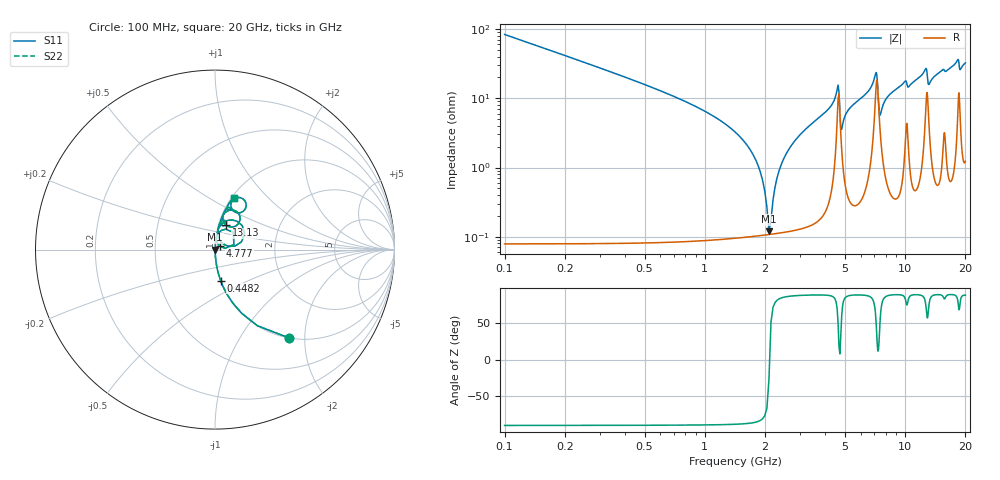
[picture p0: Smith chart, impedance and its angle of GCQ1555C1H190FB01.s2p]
!Murata Part Number: GCQ1555C1H190FB01
!These Parameters are Measured in Series Mode Connection
!Data Generated on Mar 13, 2026
!  o--ll--o
!Port1  Port2
!  o------o
!Operation Temp=25[degC], DC Bias Voltage=0[V]
!Freq. Start=100[MHz] Stop=20[GHz] 401[Steps]
# Hz S RI R 50
!Freq.(Hz) S11(Real) S11(Imag) S21(Real) S21(Imag) S12(Real) S12(Imag) S22(Real) S22(Imag)
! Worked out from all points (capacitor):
!   401 points, 100 MHz to 20 GHz, reference 50 ohm
!   read as one part in series: C = 19 pF near 199.5 MHz
!   lowest |Z| = 120 mohm at 2.09 GHz (marker M1)
!   series resonance near 2.104 GHz, so ESL is about 300 pH
!   S11 on the Smith chart (normalised r, x): 100 MHz: 1.00, -1.67; 448.2 MHz: 1.00, -0.36; 4.777 GHz: 1.06, +0.04; 13.13 GHz: 1.09, +0.30; 20 GHz: 1.02, +0.65
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1e8  0.4113 -0.4916  0.5887 0.4916  0.5887 0.4916  0.4113 -0.4916
4.4825e8  0.0316 -0.1727  0.9684 0.1727  0.9684 0.1727  0.0316 -0.1727
1.64225e9  0.00139 -0.02  0.9986 0.02  0.9986 0.02  0.00139 -0.02
1.84125e9  0.00114 -0.0107  0.9989 0.0107  0.9989 0.0107  0.00114 -0.0107
2.09e9  0.00107 -0.000543  0.9989 0.000543  0.9989 0.000543  0.00107 -0.000543
2.53775e9  0.0014 0.0154  0.9986 -0.0154  0.9986 -0.0154  0.0014 0.0154
3.43325e9  0.00335 0.0432  0.9966 -0.0432  0.9966 -0.0432  0.00335 0.0432
4.5775e9  0.0592 0.1139  0.9408 -0.1139  0.9408 -0.1139  0.0592 0.1139
4.7765e9  0.0291 0.0183  0.9709 -0.0183  0.9709 -0.0183  0.0291 0.0183
4.876e9  0.013 0.0392  0.987 -0.0392  0.987 -0.0392  0.013 0.0392
5.274e9  0.00823 0.0702  0.9918 -0.0702  0.9918 -0.0702  0.00823 0.0702
6.7665e9  0.0333 0.1387  0.9667 -0.1387  0.9667 -0.1387  0.0333 0.1387
7.1645e9  0.1514 0.134  0.8486 -0.134  0.8486 -0.134  0.1514 0.134
7.51275e9  0.0332 0.0445  0.9668 -0.0445  0.9668 -0.0445  0.0332 0.0445
8.20925e9  0.0161 0.1042  0.9839 -0.1042  0.9839 -0.1042  0.0161 0.1042
1.005e10  0.0541 0.1626  0.9459 -0.1626  0.9459 -0.1626  0.0541 0.1626
1.039825e10  0.0376 0.1369  0.9624 -0.1369  0.9624 -0.1369  0.0376 0.1369
1.2637e10  0.1066 0.2186  0.8934 -0.2186  0.8934 -0.2186  0.1066 0.2186
1.31345e10  0.0637 0.1354  0.9363 -0.1354  0.9363 -0.1354  0.0637 0.1354
1.338325e10  0.0461 0.1621  0.9539 -0.1621  0.9539 -0.1621  0.0461 0.1621
1.67165e10  0.0738 0.25  0.9262 -0.25  0.9262 -0.25  0.0738 0.25
2e10  0.1043 0.2873  0.8957 -0.2873  0.8957 -0.2873  0.1043 0.2873
